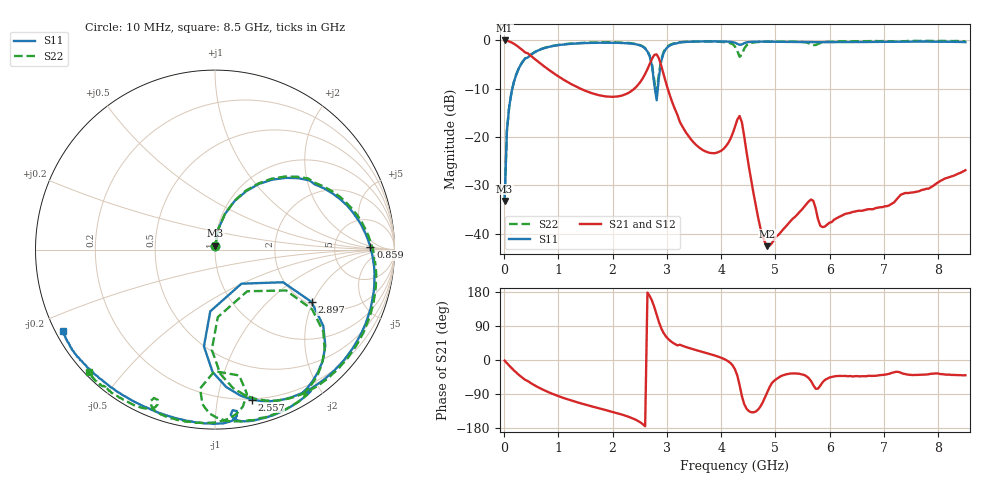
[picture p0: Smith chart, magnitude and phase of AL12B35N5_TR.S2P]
!AVX CORPORATION
!PART NUMBER AL12B35N5_TR
!DESCRIPTION: AIR CORE INDUCTOR, 35.5nH, 9 TURNS
!Agilent Technologies,E5071C,MY46102230,A.09.54
!Date: Mon Sep 03 16:01:03 2012
!Data & Calibration Information:
!Freq	S11:SOLT2(ON)	S21:SOLT2(ON)	S12:SOLT2(ON)	S22:SOLT2(ON)
# Hz S RI R 50
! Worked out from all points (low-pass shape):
!   201 points, 10 MHz to 8.5 GHz, reference 50 ohm
!   highest |S21| = -0.01 dB at 10 MHz (marker M1); lowest = -42.5 dB at 4.849 GHz (marker M2)
!   |S21| within 3 dB of the highest: start of sweep to 475.2 MHz; 2.768 GHz to 2.817 GHz (49.58 MHz wide, 1.78 % of centre)
!   lowest |S11| = -33.2 dB at 10 MHz (marker M3), VSWR 1.04, Z = 50.1 + j2.19 ohm
!   |S11| at or under -10 dB: start of sweep to 152 MHz; 2.779 GHz to 2.833 GHz (53.04 MHz wide, 1.89 % of centre)
!   |S22| runs from -33.1 to -0.1 dB; largest |S21 - S12| = 0.013
!   S11 on the Smith chart (normalised r, x): 10 MHz: 1.00, +0.04; 859 MHz: 14, +2; 2.557 GHz: 0.20, -1.25; 2.897 GHz: 2.10, -1.95; 8.5 GHz: 0.02, -0.25
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1e7  0.00171 0.0219  0.9979 -0.028  0.9903 -0.017  0.00166 0.022
5.245e7  0.0187 0.1147  0.9806 -0.1428  0.9829 -0.1423  0.0185 0.1155
1.798e8  0.174 0.3258  0.8218 -0.4213  0.8231 -0.4225  0.1717 0.3283
4.345e8  0.5558 0.3635  0.4172 -0.607  0.4175 -0.6085  0.5494 0.3749
8.59e8  0.8661 0.0148  0.0218 -0.4803  0.0215 -0.4806  0.8673 0.0414
1.4533e9  0.828 -0.4374  -0.1353 -0.2774  -0.1355 -0.2774  0.8483 -0.4099
2.557e9  0.2039 -0.8353  -0.4001 -0.075  -0.4003 -0.0749  0.2343 -0.8342
2.7268e9  -0.0616 -0.5393  -0.5912 0.2628  -0.5913 0.2633  -0.0178 -0.5575
2.8117e9  0.1476 -0.1899  -0.3513 0.6238  -0.3513 0.6243  0.1795 -0.232
2.85415e9  0.379 -0.1819  -0.1096 0.6401  -0.1094 0.6403  0.3961 -0.2278
2.8966e9  0.5379 -0.2914  0.0613 0.5426  0.0618 0.5429  0.5416 -0.3332
3.1513e9  0.5143 -0.7718  0.1436 0.1288  0.1439 0.1285  0.5089 -0.7851
3.5758e9  0.3857 -0.8951  0.0724 0.0331  0.0724 0.0331  0.3403 -0.9135
4.0003e9  0.2202 -0.9509  0.0719 0.00753  0.0719 0.00741  0.1233 -0.9563
4.255e9  0.1029 -0.9406  0.1162 -0.0533  0.1162 -0.0534  -0.0703 -0.861
4.38235e9  0.1217 -0.8999  -0.0139 -0.1413  -0.0139 -0.1412  0.135 -0.7013
4.72195e9  -0.00817 -0.971  -0.00633 -0.00968  -0.00629 -0.00961  -0.0163 -0.9643
4.8493e9  -0.0598 -0.9681  0.00069 -0.00743  0.000621 -0.00756  -0.0769 -0.9651
5.6983e9  -0.3688 -0.885  0.00874 -0.0201  0.00868 -0.02  -0.3402 -0.8268
5.8681e9  -0.424 -0.8601  0.00605 -0.0101  0.00591 -0.00983  -0.3531 -0.8852
7.09915e9  -0.7074 -0.6596  0.0159 -0.0117  0.0159 -0.0116  -0.606 -0.772
8.5e9  -0.8458 -0.4523  0.0348 -0.0293  0.0344 -0.0292  -0.7041 -0.6827
